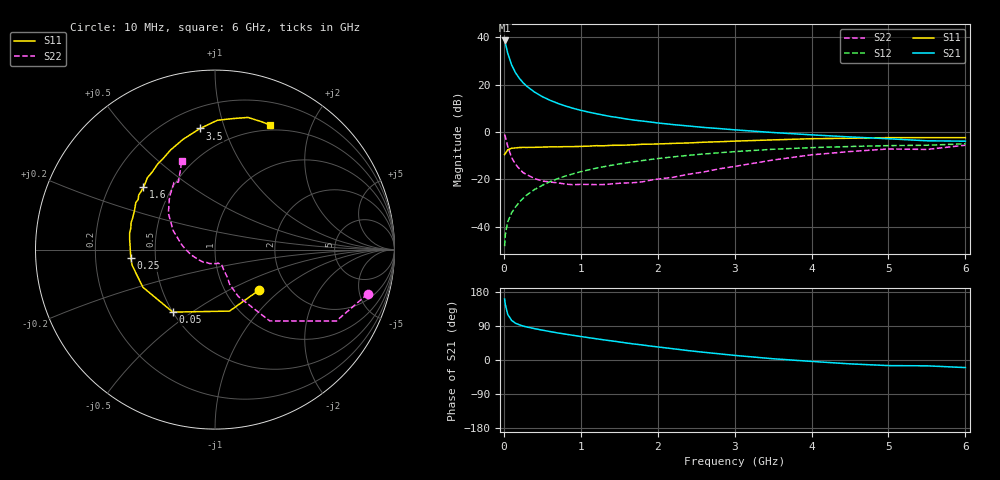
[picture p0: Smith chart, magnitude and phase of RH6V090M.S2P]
! SIEMENS Small Signal Semiconductors
! BFR106
! Si NPN RF Bipolar Junction Transistor in SOT23
! VCE = 6 V  IC = 90 mA
! Common Emitter S-Parameters:  August  1996
# GHz  S  MA  R  50
!  f  S11  S21  S12  S22
! GHz  MAG  ANG  MAG  ANG  MAG  ANG  MAG  ANG
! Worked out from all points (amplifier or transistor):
!   36 points, 10 MHz to 6 GHz, reference 50 ohm
!   highest |S21| = 38.6 dB at 10 MHz (marker M1)
!   |S21| within 3 dB of that: start of sweep to 33.2 MHz
!   unconditionally stable (mu >= 1): 193.6 MHz to 2.403 GHz
!   at 250 MHz: K = 1.04, MAG = 23.1 dB, |S12| = -28.0 dB
!   at 1.4 GHz: K = 1.06, MAG = 8.7 dB, |S12| = -14.0 dB
!   at 6 GHz: K = 0.99, MSG = 0.6 dB, |S12| = -5.0 dB
!   S11 on the Smith chart (normalised r, x): 10 MHz: 1.43, -0.73; 50 MHz: 0.50, -0.42; 250 MHz: 0.36, -0.04; 1.6 GHz: 0.35, +0.33; 3.5 GHz: 0.33, +0.83; 6 GHz: 0.44, +1.44
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0.01  0.333 -43.0  85.07 160.9  0.0039 78.7  0.8856 -16.2
0.02  0.3521 -76.7  74.17 146.0  0.0069 67.3  0.7844 -30.5
0.05  0.4201 -124.0  46.2 120.5  0.0126 59.8  0.5009 -52.5
0.1  0.453 -152.4  26.2 104.8  0.0196 63.6  0.2917 -63.6
0.15  0.4602 -163.9  17.93 97.2  0.0259 67.2  0.2096 -67.1
0.2  0.4698 -169.4  13.64 93.0  0.033 70.8  0.1685 -65.9
0.25  0.4719 -174.3  10.94 89.5  0.0398 72.0  0.1389 -66.4
0.3  0.4712 -177.4  9.162 87.1  0.0472 73.2  0.1255 -66.7
0.4  0.4739 177.1  6.929 82.8  0.0612 73.3  0.104 -66.4
0.5  0.479 173.1  5.556 78.8  0.0748 73.3  0.0924 -66.2
0.6  0.4847 168.9  4.657 75.1  0.0894 72.7  0.088 -68.5
0.7  0.4841 165.6  4.017 71.4  0.1034 71.9  0.0844 -71.9
0.9  0.4912 159.3  3.157 65.1  0.1312 69.4  0.077 -77.2
1.1  0.5019 152.8  2.627 59.0  0.1587 67.0  0.0783 -88.4
1.3  0.5108 146.9  2.253 53.1  0.1853 64.2  0.0778 -98.0
1.6  0.5289 139.0  1.87 44.7  0.2244 59.8  0.0841 -116.1
2.2  0.5736 123.9  1.43 29.7  0.2985 51.0  0.1106 -151.5
2.8  0.6217 110.1  1.179 16.3  0.3639 41.8  0.167 178.4
3.5  0.6801 97.0  0.972 3.3  0.4315 31.3  0.256 155.6
4.5  0.7368 82.2  0.785 -10.2  0.4931 16.7  0.3866 131.0
5.5  0.7583 70.0  0.651 -15.4  0.5242 6.9  0.428 118.4
6  0.7589 66.1  0.639 -20.0  0.5628 -0.2  0.525 110.7
